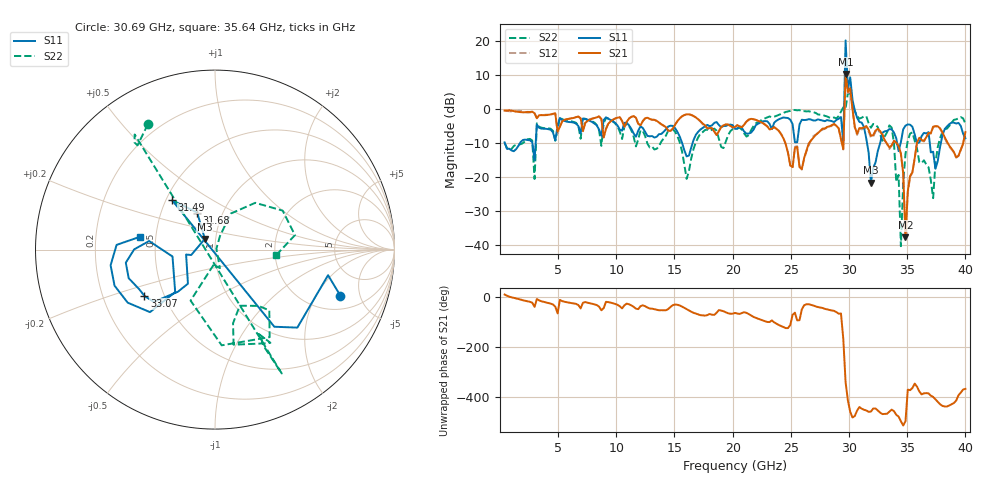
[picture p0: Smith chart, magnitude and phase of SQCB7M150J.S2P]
! Network Analyzer HP8722ES.07.66: Jul 25, 2000 Serial No. US39175408
! 26 Oct 2004  16:23:16
! Frequency  S11  S21  S12  S22
# HZ  S  DB R  50
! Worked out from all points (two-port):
!   201 points, 400 MHz to 40 GHz, reference 50 ohm
!   highest |S21| = 10.39 dB at 29.7 GHz (marker M1); lowest = -37.9 dB at 34.85 GHz (marker M2)
!   |S21| within 3 dB of the highest: 29.67722 GHz to 29.81599 GHz (138.8 MHz wide, 0.467 % of centre)
!   lowest |S11| = -21.7 dB at 31.88 GHz (marker M3), VSWR 1.18, Z = 44.4 + j5.35 ohm
!   |S11| at or under -10 dB: 418.8 MHz to 1.731 GHz (1.312 GHz wide, 122 % of centre); 31.55 GHz to 32.68 GHz (1.133 GHz wide, 3.53 % of centre); 36.94 GHz to 37.89 GHz (954.1 MHz wide, 2.55 % of centre)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
!   |S22| runs from -40.5 to 4.8 dB; largest |S21 - S12| = 2.3
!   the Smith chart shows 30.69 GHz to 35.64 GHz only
!   S11 on the Smith chart (normalised r, x): 30.69 GHz: 2.84, -3.28; 31.49 GHz: 0.54, +0.34; 31.68 GHz: 0.76, +0.33; 33.07 GHz: 0.39, -0.26; 35.64 GHz: 0.41, +0.07
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4e8  -9.82 -84.2  -0.45 10.1  -0.30 12.2  -10.03 -79.1
7.132e9  -2.75 -84.3  -6.53 -22.7  -6.45 -22.8  -3.06 -104.4
1.3666e10  -7.40 -46.0  -3.95 -52.7  -3.97 -52.5  -10.97 -76.7
2.02e10  -5.84 -12.5  -5.29 -63.3  -5.14 -62.5  -5.85 -21.6
2.4556e10  -2.57 -86.5  -10.30 -123.7  -10.27 -122.2  -0.85 -10.2
2.6932e10  -3.37 140.8  -8.43 -33.6  -7.98 -35.3  -0.91 -19.5
2.9506e10  -9.86 10.0  -11.79 -166.4  -11.93 -90.8  0.52 29.4
2.9704e10  20.26 43.2  10.39 20.2  8.72 62.8  0.13 -13.8
2.9902e10  6.05 -94.8  5.08 -52.4  4.72 -52.7  4.80 -10.8
3.01e10  9.36 -150.2  6.16 -97.8  5.92 -99.7  4.35 -45.2
3.0298e10  2.78 -177.4  0.04 -120.6  -0.20 -121.8  1.53 -61.2
3.0694e10  -2.56 -20.2  -7.26 -93.0  -7.62 -92.7  -2.03 118.2
3.1288e10  -5.32 -52.4  -5.45 -89.8  -5.75 -91.1  -2.13 124.9
3.1486e10  -8.78 131.0  -4.98 -92.5  -5.41 -93.9  -2.11 -61.7
3.1684e10  -12.81 115.7  -6.10 -98.0  -6.60 -97.7  -4.19 -63.1
3.1882e10  -21.69 133.3  -7.87 -96.8  -8.46 -94.4  -5.51 -62.5
3.307e10  -6.55 -146.7  -9.25 -106.5  -9.19 -106.1  -8.05 -52.3
3.3466e10  -5.91 -161.7  -11.33 -97.3  -11.77 -96.4  -4.81 -58.0
3.4456e10  -9.78 -133.2  -13.09 -135.4  -13.19 -135.2  -40.45 34.1
3.4852e10  -4.89 -148.7  -37.86 -135.5  -37.16 -135.1  -13.21 66.5
3.5644e10  -7.48 170.2  -14.47 14.7  -14.47 15.1  -9.34 -5.4
4e10  -8.61 -161.4  -6.78 -6.3  -6.80 -5.9  -4.24 59.0
